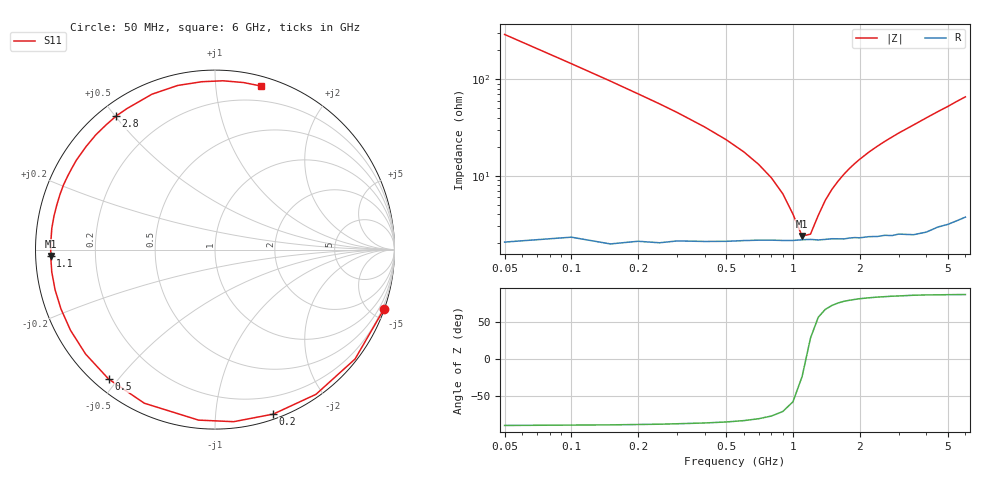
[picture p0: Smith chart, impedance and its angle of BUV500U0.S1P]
! Infineon Technologies  Discrete & RF Semiconductors
! BB 833
! Si Tuning Diode in SOD323
! VR = 0.5 V
! S-Parameters:  June  1999
# GHz  S  MA  R  50
!  f  S11
! GHz  MAG  ANG
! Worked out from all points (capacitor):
!   34 points, 50 MHz to 6 GHz, reference 50 ohm
!   read as one part to ground: C = 10.9 pF near 50 MHz
!   lowest |Z| = 2.39 ohm at 1.1 GHz (marker M1)
!   series resonance near 1.145 GHz, so ESL is about 1.8 nH
!   S11 on the Smith chart (normalised r, x): 50 MHz: 0.04, -5.82; 200 MHz: 0.04, -1.41; 500 MHz: 0.04, -0.47; 1.1 GHz: 0.04, -0.02; 2.8 GHz: 0.05, +0.50; 6 GHz: 0.07, +1.31
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0.05  0.9976 -19.5
0.1  0.9902 -38.0
0.15  0.9832 -55.1
0.2  0.9723 -70.5
0.25  0.9643 -83.8
0.3  0.9545 -95.5
0.4  0.9421 -114.7
0.5  0.9334 -129.4
0.6  0.9265 -141.1
0.7  0.9221 -150.8
0.8  0.9197 -158.9
0.9  0.9187 -165.9
1  0.9179 -172.2
1.1  0.9163 -177.8
1.3  0.917 172.6
1.4  0.9164 168.2
1.6  0.9167 160.5
1.8  0.9173 153.5
2  0.9191 147.2
2.4  0.9219 136.1
2.8  0.9258 126.5
3  0.9262 122.0
3.5  0.9343 112.1
4  0.9378 102.8
4.5  0.9382 94.5
5  0.9416 87.3
5.5  0.9442 80.3
6  0.9466 74.4
